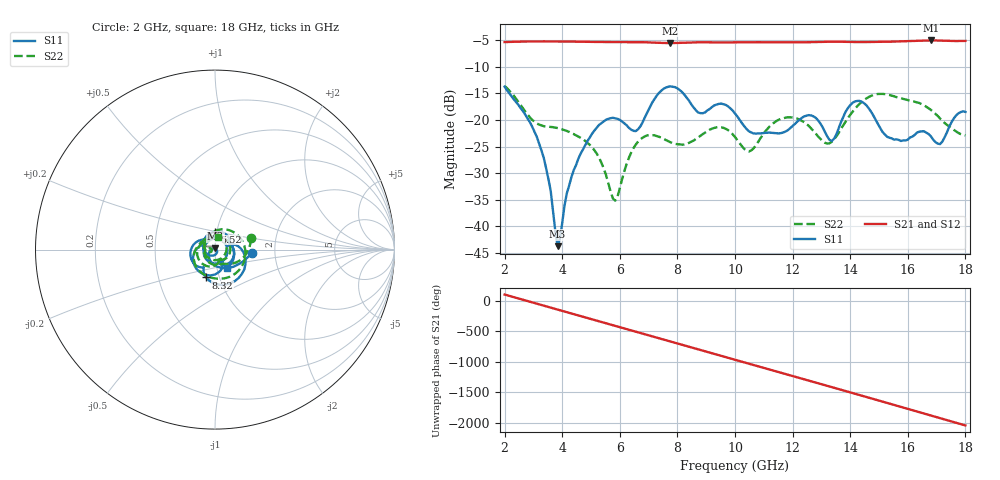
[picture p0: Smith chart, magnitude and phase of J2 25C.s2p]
!Agilent Technologies,E8363B,SG43030131,A.07.50.48
!Agilent E8363B: A.07.50.48
!Date: Wednesday, December 17, 2025 22:16:08
!Correction: S11(Full 2 Port(1,2))
!S21(Full 2 Port(1,2))
!S12(Full 2 Port(1,2))
!S22(Full 2 Port(1,2))
!S2P File: Measurements: S11, S21, S12, S22:
# Hz S  dB  R 50
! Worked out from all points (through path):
!   201 points, 2 GHz to 18 GHz, reference 50 ohm
!   highest |S21| = -5.02 dB at 16.8 GHz (marker M1); lowest = -5.5 dB at 7.76 GHz (marker M2)
!   group delay of S21, straight-line fit = 371 ps
!   lowest |S11| = -43.7 dB at 3.84 GHz (marker M3), VSWR 1.01, Z = 50.2 + j0.632 ohm
!   |S11| at or under -10 dB: start of sweep to end of sweep
!   |S22| runs from -35.2 to -13.6 dB; largest |S21 - S12| = 0.0012
!   S11 on the Smith chart (normalised r, x): 2 GHz: 1.52, -0.06; 5.52 GHz: 0.98, +0.20; 8.32 GHz: 0.87, -0.28; 18 GHz: 1.11, -0.23
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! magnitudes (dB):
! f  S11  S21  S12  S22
! 2 GHz  -13.7  -5.3  -5.3  -13.6
! 3.28 GHz  -25.7  -5.2  -5.2  -21.0
! 3.6 GHz  -33.3  -5.2  -5.2  -21.3
! 3.84 GHz  -43.7  -5.2  -5.2  -21.5
! 4.16 GHz  -33.8  -5.2  -5.2  -22.0
! 4.72 GHz  -25.5  -5.3  -5.3  -23.6
! 5.52 GHz  -19.9  -5.3  -5.3  -30.3
! 5.84 GHz  -19.7  -5.3  -5.3  -35.2
! 6.56 GHz  -22.1  -5.3  -5.3  -24.6
! 7.36 GHz  -14.9  -5.5  -5.5  -23.1
! 7.76 GHz  -13.7  -5.5  -5.5  -24.2
! 8.32 GHz  -15.8  -5.4  -5.4  -24.5
! 10 GHz  -18.8  -5.4  -5.4  -23.2
! 10.72 GHz  -22.5  -5.3  -5.3  -24.8
! 11.76 GHz  -22.1  -5.4  -5.4  -19.5
! 12.72 GHz  -19.3  -5.3  -5.3  -22.0
! 13.36 GHz  -23.9  -5.3  -5.3  -24.1
! 14.32 GHz  -16.4  -5.3  -5.3  -17.0
! 15.36 GHz  -23.3  -5.3  -5.2  -15.3
! 16.8 GHz  -23.0  -5.0  -5.0  -18.1
! 17.12 GHz  -24.5  -5.0  -5.0  -19.7
! 18 GHz  -18.5  -5.1  -5.1  -22.9
